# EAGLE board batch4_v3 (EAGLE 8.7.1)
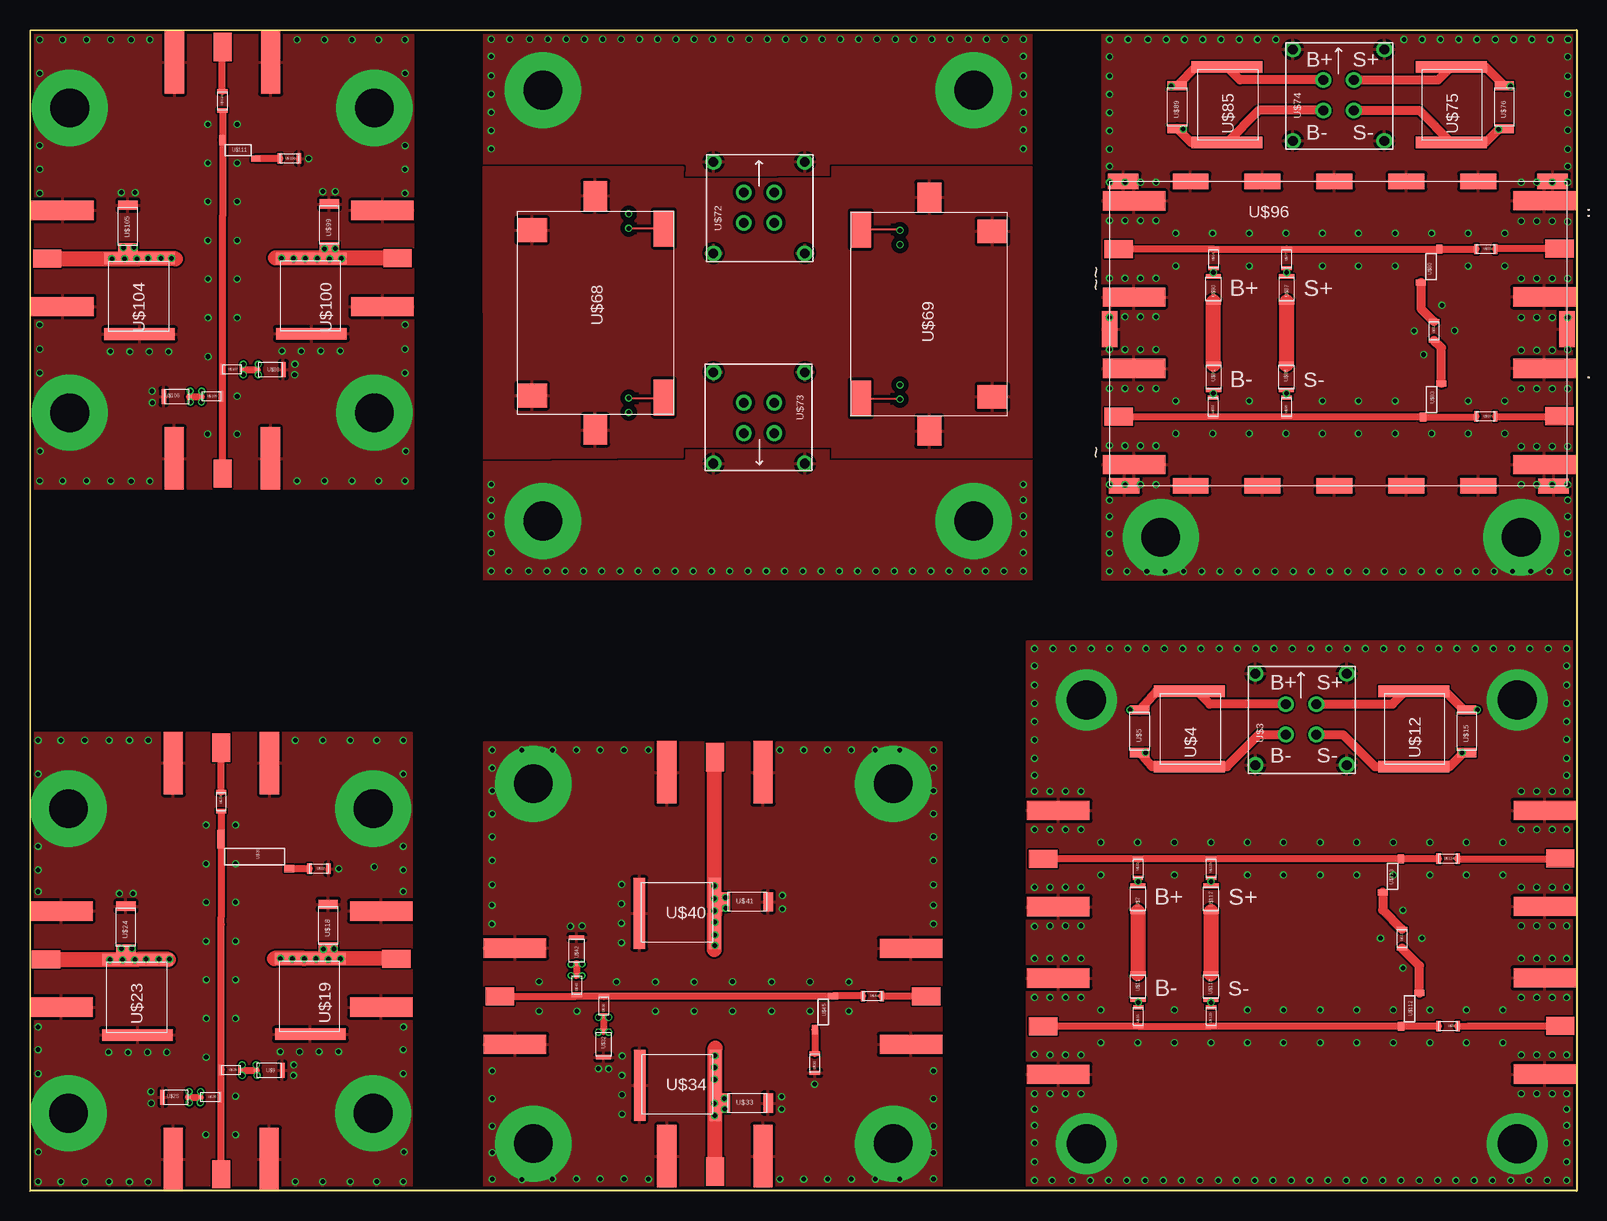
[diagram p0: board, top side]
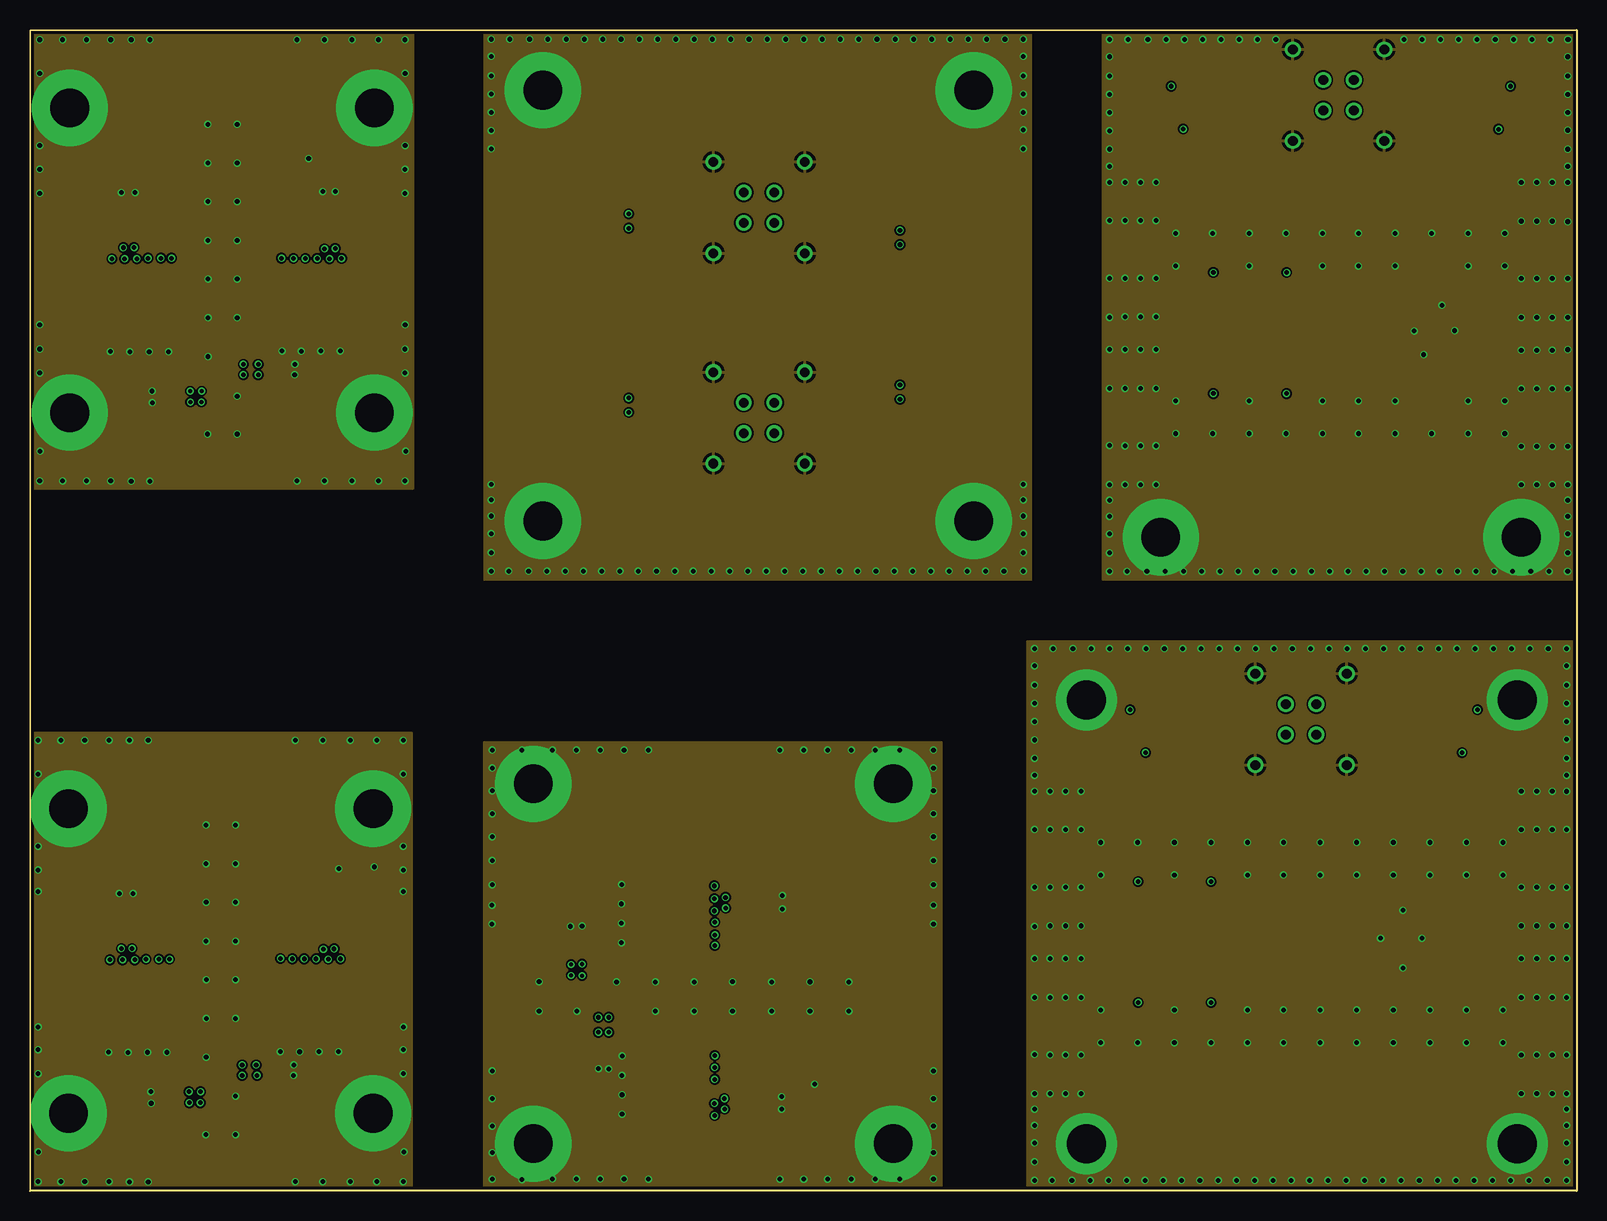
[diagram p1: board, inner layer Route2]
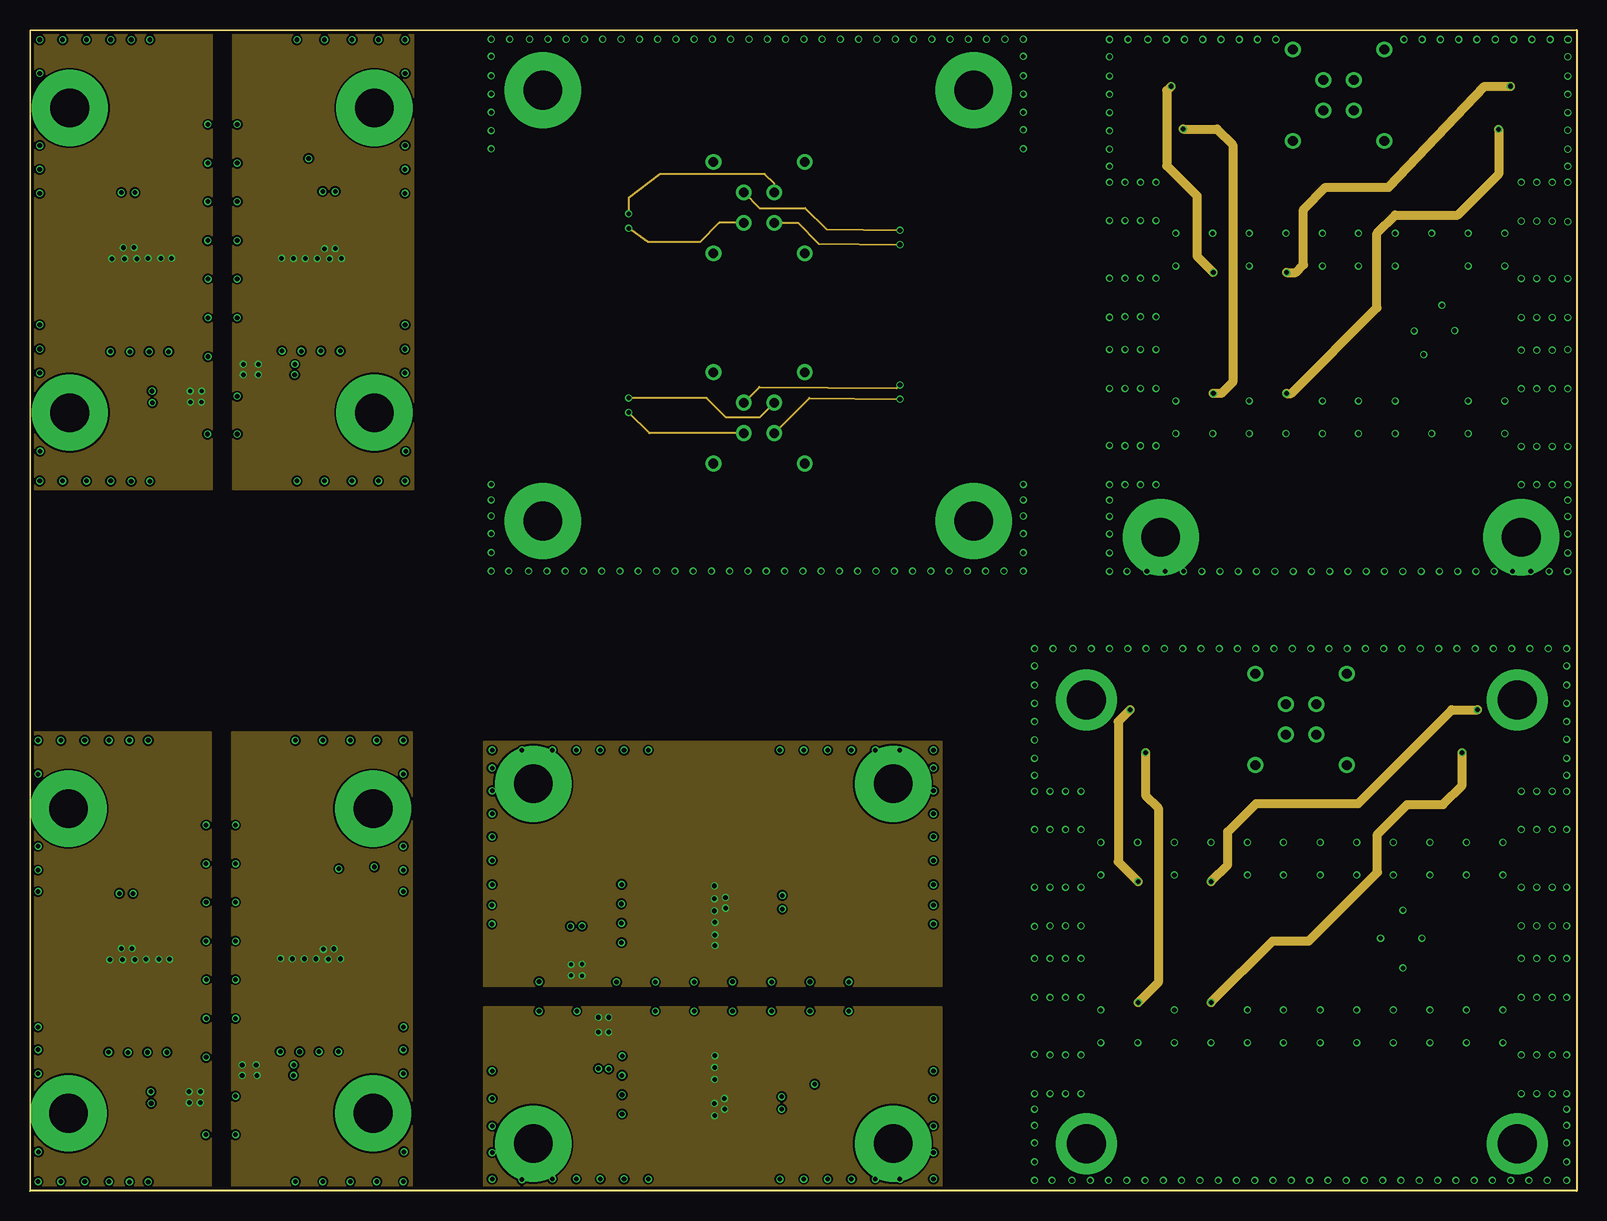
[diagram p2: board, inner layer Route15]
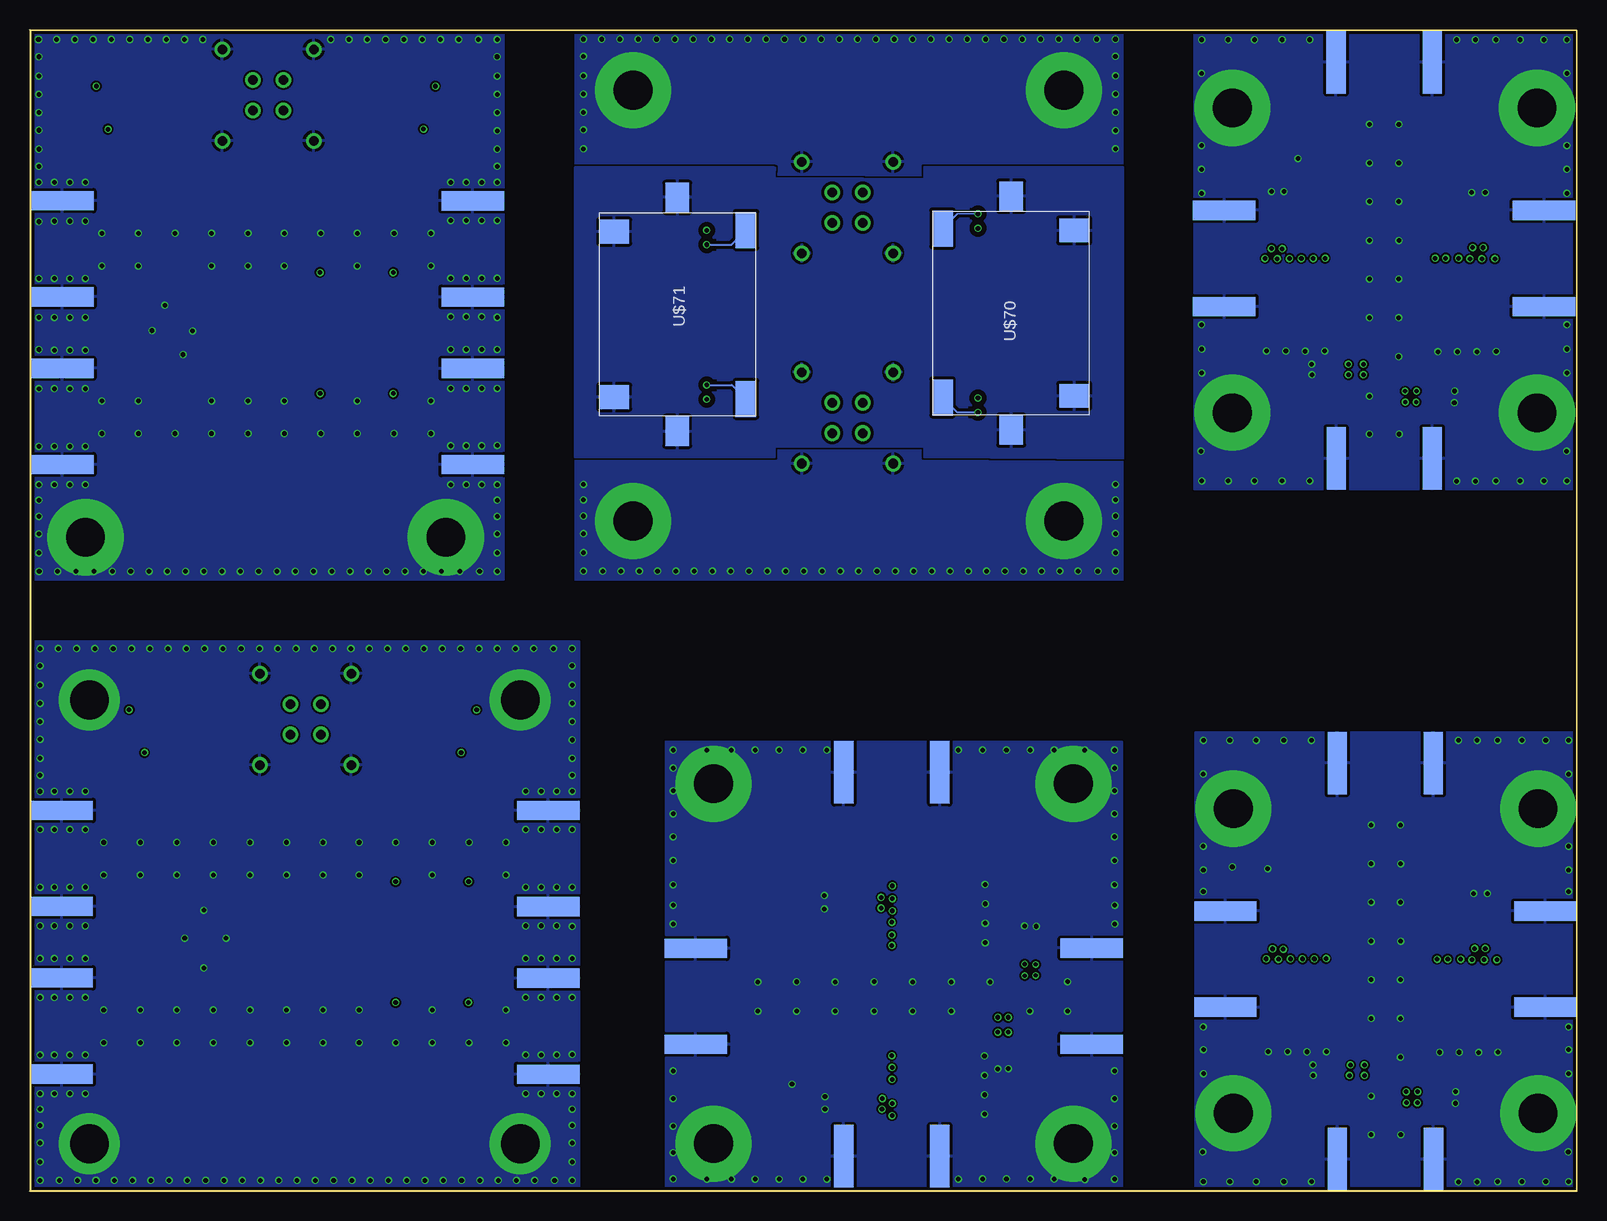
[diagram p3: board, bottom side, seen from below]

Size 128.93 x 96.77 mm. Coordinates in mm from the lower left corner, seen from the top.
Outline: 0,0 0,96.77 128.93,96.77 128.93,0 0,0
Copper layers (1*2*15*16): Top 0.01778125mm / dielectric 0.358140625mm / Route2 0.035559375mm / dielectric 28mil / Route15 0.035559375mm / dielectric 0.358140625mm / Bottom 0.01778125mm
Design rules "default *": minimum track width 6mil, minimum drill 0.35mm, track to track 6mil, track to pad 6mil, pad to pad 6mil, via to via 6mil, smd to smd 6mil, copper to edge 10mil, drill to drill 6mil, minimum pad ring 10mil, minimum via ring 4mil, stop-mask expansion 4mil, vias tented up to drill 0mil, thermal gap 10mil

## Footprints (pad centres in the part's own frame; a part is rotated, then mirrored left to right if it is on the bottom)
SMA_FEMALE = smd 1.6 x 5.207: GND_1 0.762,-2.54; GND_3 8.776,-2.54 | smd 1.6 x 5.207 bottom: GND_4 0.762,-2.54; GND_5 8.776,-2.54 | smd 1.499 x 2.362: INPUT1 4.763,-1.27
LEMO_EPG.0B.304.HLN = drill 0.8: 1 3.23,5.77; 2 5.77,5.77; 3 5.77,3.23; 4 3.23,3.23; GND1 0.69,8.31; GND2 8.31,8.31; GND3 0.69,0.69; GND4 8.31,0.69
0.47UF = smd 5.893 x 0.965: 1 2.413,-0.203; 2 2.413,6.096
.1UF = smd 1.6 x 0.762: 1 0.808,-0.206; 2 0.808,3.355
0603 = smd 0.864 x 0.356: P$1 0.396,1.565; P$2 0.396,-0.023
.03UF = smd 1.27 x 0.381: 1 0.625,-0.086; 2 0.625,2.073
ATC506WLSN = smd 1.549 x 0.635: 1 -0.762,-0.305 | smd 0.635 x 0.813: 2 1.702,5.385
ATC506WLSM = smd 0.838 x 0.508: 1 -0.381,-0.254 | smd 0.508 x 0.762: 2 1.143,2.54
LPF-B0R3+ = smd 1.981 x 2.489: GND1 1.6,1.219; GND2 15.392,1.219 | smd 2.438 x 1.981: GND3 -1.26,6.477; GND4 18.252,6.477 | smd 2.997 x 1.702: P1 1.473,12.192; P2 15.545,12.192
BMI-S-105 = smd 2.997 x 1.27: 1 30.709,25.4; 2 24.714,25.4; 3 18.72,25.4; 4 12.725,25.4; 5 6.731,25.4; 6 6.731,0.025; 7 12.725,0.029; 8 18.72,0.025; 9 24.714,0.025; 10 30.709,0.025 | smd 1.27 x 2.997: 11 -0.008,13.081; 12 38.1,13.081 | smd 2.54 x 1.27: C2 36.906,25.4; C3 1.118,25.4; C6 1.204,0.025; C7 36.982,0

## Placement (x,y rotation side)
.  SMA_FEMALESMA_FEMALE  [SMA_FEMALE]  128.78,69.33 270 top
..  SMA_FEMALESMA_FEMALE  [SMA_FEMALE]  128.78,83.3 270 top
U$1  SMA_FEMALESMA_FEMALE  [SMA_FEMALE]  83.19,22.93 90 top
U$2  SMA_FEMALESMA_FEMALE  [SMA_FEMALE]  128.83,32.48 270 top
U$3  LEMO_EPG.0B.304.HLN  [LEMO_EPG.0B.304.HLN]  110.46,34.81 90 top
U$4  0.47UF  [0.47UF]  94.24,35.57 0 top
U$5  .1UF  [.1UF]  91.7,36.73 0 top
U$6  0603  [0603]  118.99,13.33 90 top
U$7  .03UF  [.03UF]  91.73,23.35 0 top
U$8  SMA_FEMALESMA_FEMALE  [SMA_FEMALE]  0.07,14.55 90 top
U$9  .03UF  [.03UF]  18.96,10.67 270 top
U$10  0603  [0603]  92.75,27.66 180 top
U$11  .03UF  [.03UF]  92.99,18.01 180 top
U$12  0.47UF  [0.47UF]  112.93,35.57 0 top
U$13  SMA_FEMALESMA_FEMALE  [SMA_FEMALE]  128.83,18.51 270 top
U$14  SMA_FEMALESMA_FEMALE  [SMA_FEMALE]  83.19,8.96 90 top
U$15  .1UF  [.1UF]  118.96,36.73 0 top
U$16  0603  [0603]  91.99,13.74 0 top
U$17  0603  [0603]  114.77,21.78 180 top
U$18  .1UF  [.1UF]  24.05,20.53 0 top
U$19  0.47UF  [0.47UF]  25.78,19.16 180 top
U$20  SMA_FEMALESMA_FEMALE  [SMA_FEMALE]  11.19,38.21 0 top
U$21  SMA_FEMALESMA_FEMALE  [SMA_FEMALE]  20.71,0.11 180 top
U$22  SMA_FEMALESMA_FEMALE  [SMA_FEMALE]  31.82,24.08 270 top
U$23  0.47UF  [0.47UF]  11.38,19.08 180 top
U$24  .1UF  [.1UF]  7.19,20.38 0 top
U$25  .03UF  [.03UF]  13.13,7.17 90 top
U$26  0603  [0603]  17.53,9.66 90 top
U$27  0603  [0603]  24.86,26.45 90 top
U$28  0603  [0603]  15.79,7.42 90 top
U$29  0603  [0603]  16.33,33.21 180 top
U$30  ATC506WLSN  [ATC506WLSN]  16.23,28.56 270 top
U$31  SMA_FEMALESMA_FEMALE  [SMA_FEMALE]  52.33,37.43 0 top
U$32  .03UF  [.03UF]  48.45,13.21 180 top
U$33  .1UF  [.1UF]  58.18,8.12 270 top
U$34  0.47UF  [0.47UF]  56.91,6.39 90 top
U$35  SMA_FEMALESMA_FEMALE  [SMA_FEMALE]  75.99,20.98 270 top
U$36  SMA_FEMALESMA_FEMALE  [SMA_FEMALE]  37.89,11.46 90 top
U$37  SMA_FEMALESMA_FEMALE  [SMA_FEMALE]  61.87,0.34 180 top
U$38  0603  [0603]  47.44,14.64 0 top
U$39  0603  [0603]  65.03,9.87 0 top
U$40  0.47UF  [0.47UF]  56.89,20.72 90 top
U$41  .1UF  [.1UF]  58.18,24.91 270 top
U$42  .03UF  [.03UF]  44.95,19.04 0 top
U$43  0603  [0603]  45.2,16.38 0 top
U$44  0603  [0603]  71,15.84 90 top
U$45  ATC506WLSM  [ATC506WLSM]  66.57,15.98 180 top
U$68  LPF-B0R3+  [LPF-B0R3+]  40.64,81.69 270 top
U$69  LPF-B0R3+  [LPF-B0R3+]  81.45,64.59 90 top
U$70  LPF-B0R3+  [LPF-B0R3+]  40.66,64.67 90 bottom
U$71  LPF-B0R3+  [LPF-B0R3+]  81.45,81.56 270 bottom
U$72  LEMO_EPG.0B.304.HLN  [LEMO_EPG.0B.304.HLN]  65.28,77.47 90 top
U$73  LEMO_EPG.0B.304.HLN  [LEMO_EPG.0B.304.HLN]  56.28,68.94 270 top
U$74  LEMO_EPG.0B.304.HLN  [LEMO_EPG.0B.304.HLN]  113.58,86.84 90 top
U$75  0.47UF  [0.47UF]  116.06,87.6 0 top
U$76  .1UF  [.1UF]  122.09,88.76 0 top
U$77  0603  [0603]  105.14,78.48 180 top
U$80  ATC506WLSM  [ATC506WLSM]  116.34,75.97 0 top
U$81  0603  [0603]  98.24,64.56 0 top
U$82  0603  [0603]  117.44,72.46 180 top
U$83  0603  [0603]  122.12,78.11 90 top
U$84  0603  [0603]  99.05,78.48 180 top
U$85  0.47UF  [0.47UF]  97.36,87.6 0 top
U$86  0603  [0603]  104.35,64.56 0 top
U$87  .03UF  [.03UF]  104.13,74.17 0 top
U$88  .03UF  [.03UF]  105.35,68.83 180 top
U$89  .1UF  [.1UF]  94.82,88.76 0 top
U$90  .03UF  [.03UF]  98.03,74.17 0 top
U$91  .03UF  [.03UF]  99.29,68.83 180 top
U$92  0603  [0603]  122.12,64.16 90 top
U$93  ATC506WLSM  [ATC506WLSM]  117.27,67.04 180 top
U$96  BMI-S-105  [BMI-S-105]  90.02,58.75 0 top
U$97  SMA_FEMALESMA_FEMALE  [SMA_FEMALE]  0.17,72.96 90 top
U$98  .03UF  [.03UF]  19.05,69.08 270 top
U$99  .1UF  [.1UF]  24.15,78.91 0 top
U$100  0.47UF  [0.47UF]  25.87,77.54 180 top
U$101  SMA_FEMALESMA_FEMALE  [SMA_FEMALE]  11.28,96.62 0 top
U$102  SMA_FEMALESMA_FEMALE  [SMA_FEMALE]  20.81,58.52 180 top
U$103  SMA_FEMALESMA_FEMALE  [SMA_FEMALE]  31.92,82.5 270 top
U$104  0.47UF  [0.47UF]  11.55,77.52 180 top
U$105  .1UF  [.1UF]  7.36,78.81 0 top
U$106  .03UF  [.03UF]  13.22,65.58 90 top
U$107  0603  [0603]  17.62,68.07 90 top
U$108  0603  [0603]  22.4,85.66 90 top
U$109  0603  [0603]  15.89,65.83 90 top
U$110  0603  [0603]  16.42,91.63 180 top
U$111  ATC506WLSM  [ATC506WLSM]  16.28,87.2 270 top
U$112  ATC506WLSM  [ATC506WLSM]  115.44,16.24 180 top
U$113  ATC506WLSM  [ATC506WLSM]  113.14,25.14 0 top
U$114  0603  [0603]  118.99,27.28 90 top
U$115  0603  [0603]  98.84,27.66 180 top
U$116  0603  [0603]  98.05,13.74 0 top
U$117  .03UF  [.03UF]  97.83,23.35 0 top
U$118  .03UF  [.03UF]  99.05,18.01 180 top
~  SMA_FEMALESMA_FEMALE  [SMA_FEMALE]  89.48,59.78 90 top
~~  SMA_FEMALESMA_FEMALE  [SMA_FEMALE]  89.48,73.75 90 top

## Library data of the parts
. .. U$1 U$2 U$8 U$13 U$14 U$20-U$22 U$31 U$35-U$37 U$97 U$101-U$103 ~ ~~ = SMA_FEMALE
U$3 U$72-U$74 = LEMO_EPG.0B.304.HLN
U$4 U$12 U$19 U$23 U$34 U$40 U$75 U$85 U$100 U$104 = 0.47UF
U$5 U$15 U$18 U$24 U$33 U$41 U$76 U$89 U$99 U$105 = 0.1UF
U$6 U$10 U$16 U$17 U$26-U$29 U$38 U$39 U$43 U$44 U$77 U$81-U$84 U$86 U$92 U$107-U$110 U$114-U$116 = 0603
U$7 U$9 U$11 U$25 U$32 U$42 U$87 U$88 U$90 U$91 U$98 U$106 U$117 U$118 = 0.03UF
U$30 = ATC506WLSN
U$45 U$80 U$93 U$111-U$113 = ATC506WLSM
U$68-U$71 = LPF-B0R3+
U$96 = BMI-S-105

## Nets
BIAS: U$7.1 U$11.1
BIAS1: U$8.INPUT1 U$23.1 U$24.1 U$25.1 U$28.P$1
BIAS2: U$31.INPUT1 U$40.1 U$41.1 U$42.1 U$43.P$1
BIAS4: U$90.1 U$91.1
BIAS5: U$97.INPUT1 U$104.1 U$105.1 U$106.1 U$109.P$1
GND: U$1.GND_1 U$1.GND_3 U$1.GND_4 U$1.GND_5 U$2.GND_1 U$2.GND_3 U$2.GND_4 U$2.GND_5 U$3.GND1 U$3.GND2 U$3.GND3 U$3.GND4 U$13.GND_1 U$13.GND_3 U$13.GND_4 U$13.GND_5 U$14.GND_1 U$14.GND_3 U$14.GND_4 U$14.GND_5
GND1: U$8.GND_1 U$8.GND_3 U$8.GND_4 U$8.GND_5 U$9.2 U$18.2 U$19.2 U$20.GND_1 U$20.GND_3 U$20.GND_4 U$20.GND_5 U$21.GND_1 U$21.GND_3 U$21.GND_4 U$21.GND_5 U$22.GND_1 U$22.GND_3 U$22.GND_4 U$22.GND_5 U$23.2 U$24.2 U$25.2 U$27.P$2
GND2: U$31.GND_1 U$31.GND_3 U$31.GND_4 U$31.GND_5 U$32.2 U$33.2 U$34.2 U$35.GND_1 U$35.GND_3 U$35.GND_4 U$35.GND_5 U$36.GND_1 U$36.GND_3 U$36.GND_4 U$36.GND_5 U$37.GND_1 U$37.GND_3 U$37.GND_4 U$37.GND_5 U$39.P$2 U$40.2 U$41.2 U$42.2
GND4: U$68.GND1 U$68.GND2 U$68.GND3 U$68.GND4 U$69.GND1 U$69.GND2 U$69.GND3 U$69.GND4
GND5: ...GND_1 ...GND_3 ...GND_4 ...GND_5 ..GND_1 ..GND_3 ..GND_4 ..GND_5 U$74.GND1 U$74.GND2 U$74.GND3 U$74.GND4 U$96.1 U$96.2 U$96.3 U$96.4 U$96.5 U$96.6 U$96.7 U$96.8 U$96.9 U$96.10 U$96.11 U$96.12 U$96.C2 U$96.C3 U$96.C6 U$96.C7 ~.GND_1 ~.GND_3 ~.GND_4 ~.GND_5 ~~.GND_1 ~~.GND_3 ~~.GND_4 ~~.GND_5
GND8: U$97.GND_1 U$97.GND_3 U$97.GND_4 U$97.GND_5 U$98.2 U$99.2 U$100.2 U$101.GND_1 U$101.GND_3 U$101.GND_4 U$101.GND_5 U$102.GND_1 U$102.GND_3 U$102.GND_4 U$102.GND_5 U$103.GND_1 U$103.GND_3 U$103.GND_4 U$103.GND_5 U$104.2 U$105.2 U$106.2 U$108.P$2
GND9: U$70.GND1 U$70.GND2 U$70.GND3 U$70.GND4 U$71.GND1 U$71.GND2 U$71.GND3 U$71.GND4
GND10: U$72.GND1 U$72.GND2 U$72.GND3 U$72.GND4 U$73.GND1 U$73.GND2 U$73.GND3 U$73.GND4
N$1: U$21.INPUT1 U$26.P$1 U$28.P$2 U$29.P$1 U$30.1
N$2: U$1.INPUT1 U$10.P$2 U$113.2 U$114.P$1 U$115.P$2
N$3: U$17.P$1 U$112.1
N$4: U$20.INPUT1 U$29.P$2
N$5: U$27.P$1 U$30.2
N$6: U$6.P$2 U$13.INPUT1
N$7: U$36.INPUT1 U$38.P$1 U$43.P$2 U$44.P$1 U$45.1
N$8: U$35.INPUT1 U$44.P$2
N$9: U$39.P$1 U$45.2
N$20: U$68.P1 U$72.1
N$21: U$69.P2 U$72.2
N$22: U$69.P1 U$73.2
N$23: U$70.P2 U$72.3
N$24: U$71.P1 U$72.4
N$25: U$70.P1 U$73.3
N$26: U$71.P2 U$73.4
N$27: U$68.P2 U$73.1
N$28: ..INPUT1 U$92.P$2
N$29: U$82.P$1 U$93.1
N$30: U$77.P$2 U$80.2 U$83.P$1 U$84.P$2 ~~.INPUT1
N$31: U$81.P$2 U$86.P$2 U$92.P$1 U$93.2 ~.INPUT1
N$32: U$74.2 U$85.2 U$89.2
N$33: U$74.3 U$75.2 U$76.2
N$34: U$80.1 U$82.P$2
N$35: ...INPUT1 U$83.P$2
N$36: U$74.1 U$85.1 U$89.1
N$37: U$77.P$1 U$87.2
N$38: U$84.P$1 U$90.2
N$39: U$81.P$1 U$91.2
N$40: U$74.4 U$75.1 U$76.1 U$86.P$1 U$88.2
N$41: U$6.P$1 U$14.INPUT1 U$16.P$2 U$112.2 U$116.P$2
N$42: U$3.2 U$4.2 U$5.2 U$7.2 U$10.P$1
N$43: U$3.3 U$12.2 U$15.2 U$115.P$1 U$117.2
N$44: U$102.INPUT1 U$107.P$1 U$109.P$2 U$110.P$1 U$111.1
N$45: U$101.INPUT1 U$110.P$2
N$46: U$108.P$1 U$111.2
N$47: U$17.P$2 U$113.1
N$48: U$2.INPUT1 U$114.P$2
N$49: U$3.1 U$4.1 U$5.1 U$11.2 U$16.P$1
N$50: U$3.4 U$12.1 U$15.1 U$116.P$1 U$118.2
SENSE: U$117.1 U$118.1
SENSE1: U$9.1 U$18.1 U$19.1 U$22.INPUT1 U$26.P$2
SENSE2: U$32.1 U$33.1 U$34.1 U$37.INPUT1 U$38.P$2
SENSE4: U$87.1 U$88.1
SENSE5: U$98.1 U$99.1 U$100.1 U$103.INPUT1 U$107.P$2

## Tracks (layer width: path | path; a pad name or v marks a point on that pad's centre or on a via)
BIAS
  Top 0.813: 92.35,18.11 U$11.1
  Top 1.27: U$7.1 92.35,18.11
BIAS1  (via drill 0.38)
  Top 0.152: U$23.1 10.72,19.28 arc90 v10.74,19.31 | 14.21,7.79 U$28.P$1
  Top 0.2: U$25.1 13.21,8.17 arc-90 v13.25,8.26
  Top 0.592: U$24.1 U$24.1 arc90 U$24.1 | U$25.1 arc-90 13.25,7.8 arc-90 U$25.1 | U$24.1 7.99,19.72 arc90 8.43,19.28 | U$25.1 14.21,7.79
  Top 1.27: U$8.INPUT1 8.43,19.28 U$23.1 11.55,19.28
  other vias: 9.68,19.31 11.63,19.31 8.74,19.26 7.72,19.26 6.65,19.26 13.28,7.34 8.51,20.2 7.62,20.19 14.19,7.34 14.22,8.26
  pour Route15: 0.07,0.11 15.06,0.11 15.06,38.21 0.07,38.21
BIAS2  (via drill 0.35, 0.38)
  Top 0.152: 57.07,23.11 57.07,21.36 arc90 v57.1,21.33 | 45.55,17.95 45.58,17.92
  Top 0.2: 45.55,18.94 45.93,18.94 arc-90 v46.02,18.89
  Top 0.254: 45.55,17.94 arc-90 45.55,17.95 arc90 45.55,17.94 | U$43.P$1 45.55,17.94 | U$42.1 U$42.1 arc90 45.55,18.94 | U$40.1 U$40.1 arc90 57.07,23.11 | U$41.1 v57.98,24.45 arc-90 v57.98,24.45
  Top 0.592: 57.96,24.08 57.95,24.07 arc-90 57.96,24.08 | 45.55,18.94 arc-90 45.56,18.9 arc-90 45.55,18.94 | 57.96,24.08 57.51,24.08 arc90 57.07,23.64 | 45.55,18.94 45.55,17.95
  Top 1.27: 57.05,20.11 57.07,23.11 57.07,23.64 57.07,36.14 U$31.INPUT1
  other vias: 57.1,22.4 57.1,20.44 57.05,23.34 57.05,24.35 57.05,25.42 45.1,18.87 57.99,23.57 45.1,17.96 46.02,17.93
  pour Route15: 37.87,37.43 37.87,17.09 75.97,17.09 75.97,37.43
BIAS4
  Top 1.27: U$91.1 98.67,74.07 U$90.1
BIAS5  (via drill 0.35, 0.38)
  Top 0.152: U$104.1 10.89,77.72 arc90 v10.91,77.75 | 14.3,66.2 U$109.P$1
  Top 0.2: U$106.1 13.31,66.58 arc-90 v13.35,66.67
  Top 0.592: U$105.1 U$105.1 arc-90 U$105.1 | U$106.1 arc-90 13.34,66.21 arc-90 U$106.1 | U$105.1 8.16,78.16 arc90 8.6,77.72 | U$106.1 14.3,66.2
  Top 1.27: U$97.INPUT1 8.6,77.72 U$104.1 12.13,77.7
  other vias: 9.85,77.75 11.8,77.75 8.91,77.7 7.89,77.7 6.82,77.7 13.37,65.76 8.68,78.64 7.79,78.63 14.29,65.76 14.31,66.67
  pour Route15: 0.17,58.52 15.15,58.52 15.15,96.62 0.17,96.62
GND  (via drill 0.38, 3.23 pad 5.08)
  other vias: 128.09,33.3 87.61,33.3 86.32,33.3 85.03,33.3 83.74,33.3 83.74,30.11 87.61,25.3 86.32,25.3 85.03,25.3 83.74,25.3 87.61,22.09 86.32,22.09 85.03,22.09 87.61,30.11 86.32,30.11 85.03,30.11 87.61,19.36 86.32,19.36 85.03,19.36 83.74,19.36 83.74,16.12 87.61,11.33 86.32,11.33 85.03,11.33 83.74,8.09 87.61,16.12 86.32,16.12 85.03,16.12 83.74,45.21 120.47,45.21 94.56,45.21 88.46,45.21 89.99,45.21 91.51,45.21 93.04,45.21 85.29,45.21 86.94,45.21 105.23,45.21 99.13,45.21 100.66,45.21 102.18,45.21 103.7,45.21 96.08,45.21 97.61,45.21 108.28,45.21 106.75,45.21 114.37,45.21 115.9,45.21 117.42,45.21 118.94,45.21 109.8,45.21 111.32,45.21 112.85,45.21 87.61,8.09 86.32,8.09 85.03,8.09 124.31,8.09 125.6,8.09 126.89,8.09 128.09,8.09 128.09,11.33 124.31,16.12 125.6,16.12 126.89,16.12 128.09,16.12 128.09,19.36 124.31,19.36 125.6,19.36 126.89,19.36 124.31,11.33 125.6,11.33 126.89,11.33 124.31,22.09 125.6,22.09 126.89,22.09 128.09,22.09 128.09,25.3 124.31,30.11 125.6,30.11 126.89,30.11 128.09,30.11 124.31,25.3 125.6,25.3 126.89,25.3 124.31,33.3 125.6,33.3 126.89,33.3 121.99,45.21 123.52,45.21 125.04,45.21 126.56,45.21 128.09,45.21 83.74,0.86 83.74,37.59 83.74,5.46 83.74,11.37 83.74,2.41 83.74,3.98 83.74,22.04 83.74,34.64 83.74,36.06 83.74,39.11 83.74,40.64 83.74,42.16 83.74,43.77 89.26,12.35 92.35,12.35 101.49,12.35 104.5,12.35 98.44,12.35 107.55,12.35 116.69,12.35 119.74,12.35 110.59,12.35 113.64,12.35 122.79,12.35 89.26,15.07 95.39,15.07 101.49,15.07 104.5,15.07 107.55,15.07 116.69,15.07 119.74,15.07 110.59,15.07 113.64,15.07 122.79,15.07 89.26,29.04 92.35,29.04 92.32,29.04 101.49,29.04 104.5,29.04 98.44,29.04 107.55,29.04 116.69,29.04 119.74,29.04 110.59,29.04 113.64,29.04 122.79,29.04 89.26,26.33 95.39,26.33 101.49,26.33 104.5,26.33 107.55,26.33 116.69,26.33 119.74,26.33 110.59,26.33 113.64,26.33 122.79,26.33 128.09,37.65 128.09,33.3 128.09,34.64 128.09,36.06 128.09,39.11 128.09,40.64 128.09,42.16 128.09,43.77 120.38,0.86 94.47,0.86 88.38,0.86 89.9,0.86 91.43,0.86 92.95,0.86 85.2,0.86 86.85,0.86 105.14,0.86 99.05,0.86 100.57,0.86 102.09,0.86 103.62,0.86 96,0.86 97.52,0.86 108.19,0.86 106.67,0.86 114.29,0.86 115.81,0.86 117.33,0.86 118.86,0.86 109.71,0.86 111.24,0.86 112.76,0.86 121.91,0.86 123.43,0.86 124.95,0.86 126.48,0.86 128.09,0.86 128.09,5.46 128.09,2.41 128.09,3.98 116.04,21.06 114.44,18.58 114.44,23.38 112.58,21.06 83.74,6.81 128.09,6.81 95.39,29.04 95.39,12.35 88.06,3.91 123.98,3.91 88.06,40.92 123.98,40.92
  pour Route2: 83.11,0.1 83.11,45.82 128.83,45.82 128.83,0.1
  pour Top: 83.11,0.1 83.11,45.82 128.83,45.82 128.83,0.1
  pour Bottom: 83.11,0.1 83.11,45.82 128.83,45.82 128.83,0.1
GND1  (via drill 0.38, 3.23 pad 6.35)
  other vias: 25.75,26.85 28.7,27.01 7.45,24.79 8.59,24.78 10.1,7.29 10.08,8.26 21.97,9.62 21.99,10.49 3.21,6.46 3.21,31.86 28.61,6.46 28.61,31.86 0.67,0.76 0.7,3.25 0.67,9.77 0.67,11.76 0.67,13.66 0.67,24.95 0.67,26.74 0.67,28.72 0.67,34.75 0.67,37.55 31.12,24.95 31.12,26.74 31.12,28.72 31.12,34.75 31.12,0.76 31.17,3.25 31.11,9.77 31.11,11.76 31.13,13.66 2.58,0.76 4.57,0.76 6.59,0.76 8.29,0.75 22.11,0.76 24.41,0.76 26.71,0.76 28.91,0.76 2.58,37.55 4.57,37.55 6.59,37.55 8.29,37.55 9.85,37.55 22.11,37.55 24.41,37.55 26.71,37.55 28.91,37.55 31.11,37.55 9.85,0.75 14.66,4.67 14.69,11.13 14.69,14.37 14.69,17.6 14.67,20.8 14.69,24.06 14.68,27.26 14.68,30.5 17.13,4.67 17.13,7.88 17.13,14.37 17.13,17.6 17.13,20.8 17.13,24.06 17.13,27.26 9.79,11.54 8.18,11.54 6.56,11.55 11.41,11.54 17.13,30.5 24.1,11.59 22.48,11.59 20.86,11.61 25.71,11.59
  pour Route2: 31.82,0.11 0.07,0.11 0.07,38.21 31.82,38.21
  pour Top: 31.82,0.11 0.07,0.11 0.07,38.21 31.82,38.21
  pour Bottom: 31.82,0.11 0.07,0.11 0.07,38.21 31.82,38.21
GND2  (via drill 0.38, 3.23 pad 6.35)
  other vias: 65.41,8.88 62.66,6.8 62.66,7.84 62.72,24.63 62.72,23.49 45.05,22.04 46.02,22.07 47.39,10.18 48.25,10.16 38.53,31.43 41.01,36.74 47.53,36.74 49.52,36.74 51.55,36.74 62.51,36.74 64.5,36.74 66.49,36.74 72.51,36.74 75.31,31.43 62.51,0.98 64.5,0.98 66.49,0.98 72.51,0.98 38.53,0.98 41.01,0.92 47.53,0.99 49.52,0.99 51.55,0.97 38.53,29.52 38.53,27.53 38.53,25.51 38.51,23.81 38.53,9.98 38.53,7.69 38.53,5.39 38.53,3.19 75.31,29.52 75.31,27.53 75.31,25.51 75.31,23.81 75.31,22.25 75.31,9.98 75.31,7.69 75.31,5.39 75.31,3.19 75.31,0.99 38.51,22.25 41.95,33.93 71.95,33.93 41.95,3.93 71.95,3.93 42.44,17.44 48.89,17.41 52.13,17.41 55.36,17.4 58.56,17.42 61.82,17.41 65.02,17.42 68.26,17.42 42.44,14.97 45.59,14.97 52.13,14.97 55.36,14.97 58.56,14.97 61.82,14.97 65.02,14.97 49.31,22.3 49.3,23.92 49.32,25.54 49.31,20.69 68.26,14.97 49.36,8 49.35,9.62 49.37,11.24 49.36,6.39 45.54,36.74 45.54,0.99 68.48,36.74 68.48,0.98 43.56,36.74 43.56,0.99 38.53,36.74 75.31,36.74 38.53,33.34 38.53,35.25 75.31,33.34 75.31,35.25 70.47,36.74 70.47,0.98
  pour Top: 37.87,0.32 37.87,37.43 75.97,37.43 75.97,0.32
  pour Route2: 37.87,0.32 37.87,37.43 75.97,37.43 75.97,0.32
  pour Bottom: 37.87,0.32 37.87,37.43 75.97,37.43 75.97,0.32
GND4
  pour Top (isolate 0.406): 54.36,85.34 37.79,85.34 37.81,61.05 54.42,61.18 54.42,85.34 54.42,85.08
  pour Top (isolate 0.406): 66.85,61.16 83.54,61.14 83.54,85.33 66.85,85.35
  pour Top (isolate 0.254): 53.09,84.36 71.65,84.46 71.6,62 50.89,61.97 50.74,77.83 50.66,84.41
GND5  (via drill 0.38, 3.23 pad 6.35)
  other vias: 93.86,84.07 92.57,84.07 91.28,84.07 89.99,84.07 89.99,80.89 93.86,76.07 92.57,76.07 91.28,76.07 89.99,76.07 93.86,72.86 92.57,72.86 91.28,72.86 93.86,80.89 92.57,80.89 91.28,80.89 93.86,70.14 92.57,70.14 91.28,70.14 89.99,70.14 89.99,66.89 93.86,62.11 92.57,62.11 91.28,62.11 89.99,58.87 93.86,66.89 92.57,66.89 91.28,66.89 89.99,95.98 126.72,95.98 100.81,95.98 94.71,95.98 96.24,95.98 97.76,95.98 99.28,95.98 91.54,95.98 93.19,95.98 102.33,95.98 103.86,95.98 114.52,95.98 120.62,95.98 122.14,95.98 123.67,95.98 125.19,95.98 116.05,95.98 117.57,95.98 119.1,95.98 93.86,58.87 92.57,58.87 91.28,58.87 128.24,95.98 89.99,51.63 89.99,88.36 89.99,56.23 89.99,62.15 89.99,53.18 89.99,54.76 89.99,72.82 89.99,85.42 89.99,86.84 89.99,89.89 89.99,91.41 89.99,92.93 89.99,94.54 95.51,63.13 98.59,63.13 107.74,63.13 110.75,63.13 104.69,63.13 113.8,63.13 122.94,63.13 116.84,63.13 119.89,63.13 95.51,65.84 101.64,65.84 107.74,65.84 110.75,65.84 113.8,65.84 122.94,65.84 119.89,65.84 95.51,79.82 98.59,79.82 98.57,79.82 107.74,79.82 110.75,79.82 104.69,79.82 113.8,79.82 122.94,79.82 116.84,79.82 119.89,79.82 95.51,77.1 101.64,77.1 107.74,77.1 110.75,77.1 113.8,77.1 122.94,77.1 119.89,77.1 126.63,51.63 100.72,51.63 94.63,51.63 96.15,51.63 97.67,51.63 99.2,51.63 91.45,51.63 93.1,51.63 111.39,51.63 105.29,51.63 106.82,51.63 108.34,51.63 109.87,51.63 102.25,51.63 103.77,51.63 114.44,51.63 112.91,51.63 120.53,51.63 122.06,51.63 123.58,51.63 125.11,51.63 115.96,51.63 117.49,51.63 119.01,51.63 128.15,51.63 118.75,71.71 116.17,69.71 117.69,73.83 115.38,71.69 89.99,57.58 101.64,79.82 101.64,63.13 128.19,84.07 128.19,58.87 128.19,70.14 128.19,95.98 128.19,88.42 128.19,84.07 128.19,85.42 128.19,86.84 128.19,89.89 128.19,91.41 128.19,92.93 128.19,94.54 128.19,51.63 128.19,56.23 128.19,53.18 128.19,54.76 128.19,57.58 124.31,58.87 125.6,58.87 126.9,58.87 128.19,58.87 128.19,62.06 124.31,66.87 125.6,66.87 126.9,66.87 128.19,66.87 124.31,70.08 125.6,70.08 126.9,70.08 124.31,62.06 125.6,62.06 126.9,62.06 124.31,72.8 125.6,72.8 126.9,72.8 128.19,72.8 128.19,76.05 124.31,80.83 125.6,80.83 126.9,80.83 128.19,84.07 124.31,76.05 125.6,76.05 126.9,76.05 124.31,84.07 125.6,84.07 126.9,84.07 128.19,80.79 128.19,70.13 94.26,54.48 124.31,54.48
  pour Top: 89.41,50.93 89.41,96.65 128.78,96.65 128.78,50.93
  pour Route2: 89.41,50.93 89.41,96.65 128.78,96.65 128.78,50.93
  pour Bottom: 89.41,50.93 89.41,96.65 128.78,96.65 128.78,50.93
GND8  (via drill 0.38, 3.23 pad 6.35)
  other vias: 23.23,86.07 25.44,83.31 24.4,83.31 7.62,83.23 8.76,83.22 10.2,65.7 10.17,66.67 22.06,68.04 22.08,68.9 0.81,59.18 0.85,61.66 0.81,68.18 0.81,70.17 0.81,72.2 0.81,83.16 0.81,85.15 0.81,87.14 0.81,93.16 0.81,95.96 31.26,83.16 31.27,85.15 31.27,87.14 31.27,93.16 31.26,59.18 31.32,61.66 31.26,68.18 31.26,70.17 31.27,72.2 2.72,59.18 4.71,59.18 6.73,59.18 8.44,59.16 22.26,59.18 24.55,59.18 26.85,59.18 29.05,59.18 2.72,95.96 4.71,95.96 6.73,95.96 8.44,95.96 10,95.96 22.26,95.96 24.55,95.96 26.85,95.96 29.05,95.96 31.26,95.96 10,59.16 3.31,64.87 3.31,90.27 28.71,64.87 28.71,90.27 14.8,63.09 14.83,69.54 14.84,72.78 14.84,76.01 14.82,79.21 14.83,82.47 14.82,85.67 14.83,88.91 17.27,63.09 17.27,66.25 17.27,72.78 17.27,76.01 17.27,79.21 17.27,82.47 17.27,85.67 9.94,69.96 8.32,69.95 6.7,69.97 11.56,69.96 17.27,88.91 24.24,70.01 22.62,70 21,70.02 25.86,70.01
  pour Route2: 31.92,58.52 0.17,58.52 0.17,96.62 31.92,96.62
  pour Top: 31.92,58.52 0.17,58.52 0.17,96.62 31.92,96.62
  pour Bottom: 31.92,58.52 0.17,58.52 0.17,96.62 31.92,96.62
GND9
  pour Bottom (isolate 0.406): 66.91,85.32 83.53,85.32 83.53,61.16 66.85,61.16 66.85,85.32 66.85,85.06
  pour Bottom (isolate 0.406): 54.42,61.19 37.8,61.04 37.78,85.33 54.41,85.33
  pour Bottom (isolate 0.254): 68.2,84.47 50.66,84.39 50.89,61.98 71.59,62 71.62,84.47 68.27,84.39
GND10  (via drill 0.38, 3.23 pad 6.35)
  other vias: 38.45,58.89 38.45,96.01 75.18,96.01 49.27,96.01 43.17,96.01 44.7,96.01 46.22,96.01 47.74,96.01 40,96.01 41.65,96.01 59.94,96.01 53.84,96.01 55.36,96.01 56.89,96.01 58.41,96.01 50.79,96.01 52.32,96.01 62.98,96.01 61.46,96.01 69.08,96.01 70.6,96.01 72.13,96.01 73.65,96.01 64.51,96.01 66.03,96.01 67.56,96.01 82.8,58.89 76.7,96.01 78.22,96.01 79.75,96.01 81.27,96.01 82.8,96.01 38.45,51.66 38.45,88.39 38.45,56.25 38.45,53.21 38.45,54.78 38.45,86.86 38.45,89.91 38.45,91.43 38.45,92.96 38.45,94.57 82.8,88.44 82.8,86.86 82.8,89.91 82.8,91.43 82.8,92.96 82.8,94.57 75.09,51.66 49.18,51.66 43.09,51.66 44.61,51.66 46.13,51.66 47.66,51.66 39.91,51.66 41.56,51.66 59.85,51.66 53.75,51.66 55.28,51.66 56.8,51.66 58.33,51.66 50.71,51.66 52.23,51.66 62.9,51.66 61.37,51.66 68.99,51.66 70.52,51.66 72.04,51.66 73.57,51.66 64.42,51.66 65.95,51.66 67.47,51.66 76.61,51.66 78.14,51.66 79.66,51.66 81.19,51.66 82.8,51.66 82.8,56.25 82.8,53.21 82.8,54.78 38.45,57.6 82.8,57.6 42.75,55.83 78.66,55.83 42.75,91.74 78.66,91.74
  pour Top (rank 5): 37.8,50.93 37.8,96.65 83.52,96.65 83.52,50.93
  pour Route2 (rank 5): 37.8,50.93 83.52,50.93 83.52,96.65 37.8,96.65
  pour Bottom (rank 5): 37.8,50.93 37.8,96.65 83.52,96.65 83.52,50.93
N$1
  Top 0.152: U$28.P$2 15.95,7.68 U$21.INPUT1 15.95,29.14 | U$26.P$1 15.96,10.07 15.95,10.09 | 15.95,28.75 15.95,29.14 | 15.95,29.29 15.95,31.53 15.95,31.63 U$29.P$1 | 15.95,28.44 15.95,28.17 | U$30.1 15.95,29.29 | 15.95,29.29 15.95,29.14
  Top 0.592: 15.95,22.2 15.95,22.85 | 15.95,31.53 15.95,31.52 | 15.95,31.52 15.95,29.14 15.95,28.44 15.95,22.85 | 15.96,31.53 15.95,31.52 | U$21.INPUT1 15.95,10.09 15.95,22.85
N$2
  Top 0.254: U$115.P$2 98.44,27.66 | U$10.P$2 92.45,27.68 92.48,27.65
  Top 0.584: U$1.INPUT1 84.49,27.65 92.48,27.65 98.44,27.66 U$113.2 U$114.P$1
N$3
  Top 0.762: U$112.1 115.82,18.77 U$17.P$1
N$4
  Top 0.152: 15.93,36.29 15.95,36.3
  Top 0.592: 15.93,36.07 15.82,36.17 15.95,36.3 U$20.INPUT1 | U$29.P$2 15.93,36.29
N$5
  Top 0.584: U$27.P$1
  Top 0.592: U$27.P$1 U$30.2
N$6
  Top 0.584: U$6.P$2 119.87,13.74 U$13.INPUT1
N$7
  Top 0.254: U$43.P$2 45.6,16.32 arc-90 45.48,16.2
  Top 0.592: U$36.INPUT1 45.46,16.22 arc90 45.48,16.2 U$38.P$1 arc-90 47.87,16.23 U$45.1 arc-90 U$45.1 U$44.P$1
N$8
  Top 0.592: U$44.P$2 74.7,16.23 arc-90 U$35.INPUT1
N$9
  Top 0.592: U$45.2 U$39.P$1 | U$39.P$1 arc-90 U$39.P$1
N$20  (via drill 0.38)
  Top 0.178: v49.91,80.25 52.81,80.24 U$68.P1
  Route15 0.178: U$72.1 57.46,80.7 55.86,79.1 51.52,79.1 v49.91,80.25
N$21  (via drill 0.38)
  Top 0.178: v72.52,80.07 72.46,80.14 U$69.P2
  Route15 0.178: U$72.2 60.81,81.94 64.62,81.94 66.39,80.17 v72.52,80.07
N$22  (via drill 0.38)
  Top 0.178: U$69.P1 69.18,65.99 v72.52,65.99
  Route15 0.178: U$73.2 64.98,66.09 v72.52,65.99
N$23  (via drill 0.38)
  Route15 0.178: U$72.3 62.05,83.95 61.24,84.76 52.52,84.76 49.9,82.77 49.9,81.46 v49.91,81.44
  Bottom 0.178: 53.22,80.22 U$70.P2 | U$70.P2 | v49.91,81.44 51.64,81.43 U$70.P2
N$24  (via drill 0.38)
  Route15 0.178: U$72.4 64,80.7 65.72,78.98 v72.52,78.88
  Bottom 0.178: 68.71,80.09 U$71.P1 70.47,78.88 v72.52,78.88
N$25  (via drill 0.38)
  Route15 0.178: U$73.3 51.64,63.17 v49.91,64.9
  Bottom 0.178: v49.91,64.9 51.6,64.9 U$70.P1
N$26  (via drill 0.38)
  Route15 0.178: U$73.4 60.81,67 72.24,66.9 v72.52,67.18
  Bottom 0.178: 68.73,66.02 U$71.P2 70.42,67.18 v72.52,67.18
N$27  (via drill 0.38)
  Top 0.178: v49.91,66.09 52.78,66.09 U$68.P2
  Route15 0.178: U$73.1 60.81,64.47 58.04,64.47 56.41,66.09 v49.91,66.09
N$28
  Top 0.584: U$92.P$2 128.18,64.55 | 128.18,64.55 128.22,64.52 | 128.18,64.55 128.16,64.57 ..INPUT1
N$29
  Top 0.762: U$93.1 117.65,70.28 U$82.P$1
N$30
  Top 0.584: ~~.INPUT1 90.76,78.5 U$84.P$2 U$77.P$2 U$80.2 U$83.P$1
N$31
  Top 0.584: ~.INPUT1 98.69,64.54 U$81.P$2 U$86.P$2 116.09,64.54 U$93.2 120.51,64.5 U$92.P$1
N$32  (via drill 0.38)
  Top 0.343: U$89.2 95.59,92.08 v95.13,92.08
  Top 0.762: U$74.2 100.86,92.61 U$85.2 97.2,93.69 U$89.2
  Route15 0.762: v95.13,92.08 94.77,91.72 94.77,85.45 97.28,82.94 97.28,77.93 v98.64,76.56
N$33  (via drill 0.38)
  Top 0.343: U$76.2 122.93,92.08 v123.41,92.08
  Top 0.762: U$74.3 117.39,92.61 U$75.2 121.32,93.69 U$76.2
  Route15 0.762: v104.75,76.56 105.52,76.56 106.15,77.2 106.15,81.81 107.99,83.65 113.25,83.65 121.26,92.08 v123.41,92.08
N$34
  Top 0.762: U$80.1 115.95,73.56 U$82.P$2
N$35
  Top 0.584: ...INPUT1 122.18,78.54 U$83.P$2
N$36  (via drill 0.38)
  Top 0.343: U$89.1 95.67,88.51 v96.13,88.51
  Top 0.762: U$74.1 102.45,90.07 U$85.1 96.79,87.39 U$89.1
  Route15 0.762: v98.64,66.47 99.31,66.47 100.25,67.41 100.25,87.21 98.95,88.51 v96.13,88.51
N$37
  Top 0.254: U$77.P$1 U$87.2
N$38
  Top 0.254: U$84.P$1 U$90.2
N$39
  Top 0.254: U$91.2 98.64,66.73 U$81.P$1
N$40  (via drill 0.38)
  Top 0.254: U$88.2 104.73,66.15 U$86.P$1 | U$76.1 122.48,88.56 v122.42,88.5
  Top 0.343: v104.75,66.47 104.75,66.74 U$88.2
  Top 0.762: U$74.4 115.79,90.07 U$75.1 121.32,87.39 v122.42,88.5
  Route15 0.762: v122.42,88.5 122.42,84.76 119.01,81.35 113.8,81.35 112.27,79.83 112.27,73.61 105.13,66.47 v104.75,66.47
N$41
  Top 0.152: U$116.P$2 98.48,13.72 98.49,13.71
  Top 0.584: U$14.INPUT1 84.18,13.71 U$16.P$2 98.49,13.71 98.49,13.72 | 98.49,13.72 U$112.2 114.32,13.73 U$6.P$1 | 98.52,13.74 98.49,13.72
N$42  (via drill 0.38)
  Top 0.152: 96.93,41.66 97.27,41.65 | U$10.P$1
  Top 0.254: U$5.2 92.36,40.1 v91.7,40.1 | 92.37,26.08 U$10.P$1 92.36,25.49 U$7.2 | v92.37,25.78 U$10.P$1 | U$4.2 96.92,41.66 96.93,41.66
  Top 0.762: U$4.2 93.95,41.66 U$5.2 | U$3.2 98.34,40.58 97.27,41.65
  Route15 0.762: v91.7,40.1 90.72,39.12 90.72,27.43 v92.37,25.78
N$43  (via drill 0.38)
  Top 0.152: 114.62,41.65 114.58,41.65 114.59,41.66 114.7,41.66 | 114.63,41.66 114.7,41.66 | U$15.2 120,40.09 119.51,40.09 | 114.99,41.66 114.7,41.66 | 114.7,41.66 | U$3.3 107.2,40.58 | 107.2,40.58 | 98.43,25.97 98.43,25.89 v98.45,25.78 98.44,25.88 U$115.P$1
  Top 0.254: U$15.2 120.66,40.09 v120.67,40.09 | U$117.2 98.45,25.87 | 114.99,41.66 U$12.2 114.65,41.66 114.64,41.65 | U$3.3
  Top 0.584: 98.45,25.87 v98.45,25.78
  Top 0.762: 114.7,41.66 117.94,41.66 119.51,40.09 | U$3.3 113.57,40.58 114.64,41.65
  Route15 0.762: v98.45,25.78 99.85,27.19 99.85,29.93 102.21,32.29 110.71,32.29 118.51,40.09 v120.67,40.09
N$44
  Top 0.152: U$109.P$2 16.04,66.09 U$102.INPUT1 16.04,87.61 | U$107.P$1 16.06,68.48 16.04,68.5 | 16.04,87.16 16.04,87.59 | 16.04,87.61 16.04,89.95 16.04,90.05 U$110.P$1 | 16.04,87.61 | U$111.1 16.04,87.59 | 16.04,87.59 16.04,87.61
  Top 0.592: 16.04,80.61 16.04,81.26 | 16.04,89.95 16.04,89.93 | 16.04,89.93 16.04,87.61 16.04,81.26 | 16.05,89.94 16.04,89.93 | U$102.INPUT1 16.04,68.5 16.04,81.26
N$45
  Top 0.152: 16.03,94.7 16.04,94.71
  Top 0.592: 16.02,94.48 15.92,94.59 16.04,94.71 U$101.INPUT1 | U$110.P$2 16.03,94.7
N$46
  Top 0.152: U$108.P$1 20.82,86.06 | 18.84,86.06 U$111.2
  Top 0.592: 20.82,86.06 18.84,86.06
N$47
  Top 0.762: U$113.1 112.76,23.42 U$17.P$2
N$48
  Top 0.584: U$114.P$2 127.52,27.68 U$2.INPUT1
N$49  (via drill 0.38)
  Top 0.254: U$16.P$1 92.41,15.31 92.38,15.34 U$11.2 92.38,15.65 v92.39,15.69
  Top 0.343: U$5.1 92.38,36.53 v92.99,36.53
  Top 0.762: U$3.1 102.45,38.04 99.78,35.36 U$4.1 93.54,35.36 U$5.1
  Route15 0.343: 93.12,36.4 v92.99,36.53
  Route15 0.762: v92.99,36.53 92.99,32.98 94.05,31.92 94.05,17.36 v92.39,15.69
N$50  (via drill 0.38)
  Top 0.152: U$15.1 120,36.52 119.51,36.52 | U$3.4 107.2,38.04 | 107.2,38.04 | 114.03,35.36
  Top 0.254: U$15.1 v119.38,36.52 v119.38,36.53 | U$116.P$1 v98.45,15.69 98.43,15.72 U$118.2
  Top 0.762: 107.2,38.04 109.43,38.04 112.11,35.36 114.03,35.36 | 114.03,35.36 118.35,35.36 119.51,36.52 | U$12.1 114.03,35.36
  Route15 0.762: v98.45,15.69 103.58,20.83 106.59,20.83 112.32,26.56 112.32,29.72 114.8,32.2 117.78,32.2 119.38,33.8 v119.38,36.53
SENSE
  Top 1.27: U$117.1 98.45,18.12 U$118.1
SENSE1  (via drill 0.38)
  Top 0.152: U$19.1 20.38,19.36 arc-90 20.37,19.37 | 22.87,19.36 arc-90 22.85,19.37 arc90 22.87,19.36 | U$19.1 22.87,19.36 | U$19.1 23.82,19.36 arc-90 v23.85,19.33 | U$26.P$2 17.57,10.04 17.7,10.04
  Top 0.2: U$9.1 18.87,9.69 arc90 v18.93,9.62
  Top 0.592: 30.54,19.46 U$22.INPUT1 | U$18.1 24.86,19.79 arc-90 24.43,19.36 U$19.1 | 17.7,10.04 U$9.1 | U$9.1 arc-90 U$9.1 arc90 U$9.1 | 20.37,19.37 arc90 20.36,19.36
  Top 1.27: 30.54,19.46 arc-90 U$22.INPUT1 22.85,19.37 20.37,19.37
  other vias: 25.35,20.17 24.46,20.15 24.86,19.31 25.88,19.33 22.86,19.33 21.87,19.33 20.88,19.36 17.69,9.62 17.69,10.49 18.86,10.49
  pour Route15 (rank 2): 31.82,0.11 16.84,0.11 16.84,38.21 31.82,38.21
SENSE2  (via drill 0.38)
  Top 0.152: 47.82,14.6 47.8,14.58 47.8,14.45
  Top 0.2: 47.8,13.28 47.45,13.28 arc90 v47.39,13.22
  Top 0.254: v57.1,11.27 arc-90 57.12,11.25 U$34.1 57.12,11.87 arc90 57.1,11.88 | U$33.1 57.98,7.6 arc90 v57.88,7.69 | U$38.P$2 U$38.P$2 arc90 47.82,14.6 | U$32.1 U$32.1 arc90 47.8,13.28
  Top 0.592: 47.8,14.45 47.8,13.28 | 47.8,13.28 arc-90 47.79,13.29 arc90 47.8,13.28
  Top 1.27: U$37.INPUT1 57.1,11.88 arc-90 57.12,11.9
  other vias: 57.91,6.8 57.05,7.28 57.07,6.27 57.07,9.29 57.07,10.28 47.39,14.46 48.25,14.46 48.25,13.22
  pour Route15 (rank 2): 37.87,0.32 37.87,15.31 75.97,15.31 75.97,0.32
SENSE4
  Top 1.27: U$88.1 104.75,68.94 U$87.1
SENSE5  (via drill 0.38)
  Top 0.152: U$100.1 20.48,77.75 arc-90 20.46,77.76 | 22.96,77.75 arc-90 22.95,77.76 arc90 22.96,77.75 | U$100.1 22.96,77.75 | U$100.1 23.92,77.75 arc-90 v23.94,77.72 | U$107.P$2 17.66,68.45 17.79,68.45
  Top 0.2: U$98.1 18.96,68.1 arc90 v19.02,68.04
  Top 0.592: U$103.INPUT1 30.64,77.87 | U$99.1 24.95,78.17 arc-90 24.53,77.75 U$100.1 | 17.79,68.45 U$98.1 | U$98.1 arc-90 U$98.1 arc90 U$98.1 | 20.46,77.76 arc90 20.45,77.75
  Top 1.27: 30.64,77.87 arc90 U$103.INPUT1 22.95,77.76 20.46,77.76
  other vias: 25.44,78.56 24.55,78.53 24.96,77.7 25.97,77.72 22.95,77.72 21.96,77.72 20.97,77.75 17.78,68.04 17.78,68.9 19.03,68.9
  pour Route15 (rank 2): 31.92,58.52 16.93,58.52 16.93,96.62 31.92,96.62

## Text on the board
tPlace: B+ | S+ | B- | S- | B+ | S+ | B- | S- | B+ | S+ | B- | S- | B+ | S+ | B- | S-
tStop: Low-Pass Filter Board v2 | S. Patel | Double Ended Bias Tee v2 | B. Korzh | E. Ramirez | Single Ended | Bias-T | S. Patel | E. Ramirez | Double Ended Bias Tee v2 | B. Korzh | S. Patel | S. Patel | E. Ramirez
bStop: B. Korzh | E. Ramirez | August 2019 | August 2019 | August 2019 | August 2019 | August 2019 | August 2019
